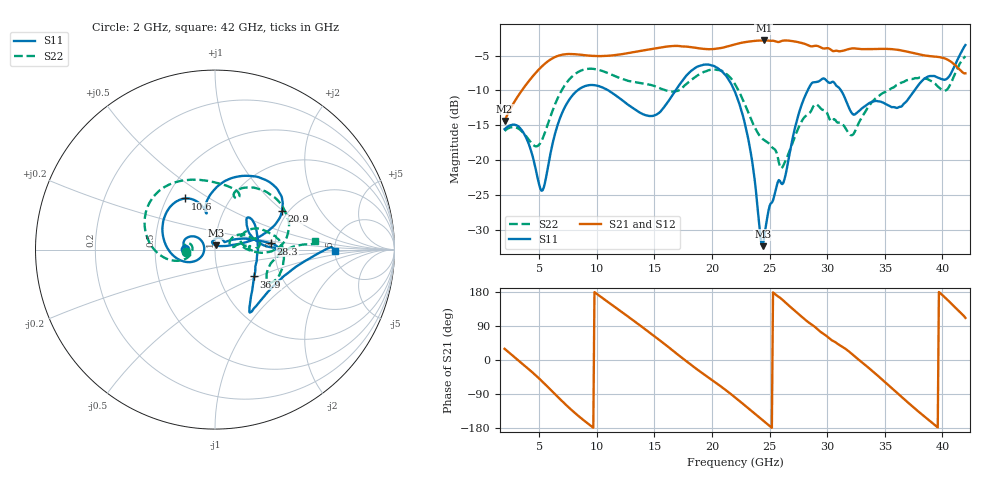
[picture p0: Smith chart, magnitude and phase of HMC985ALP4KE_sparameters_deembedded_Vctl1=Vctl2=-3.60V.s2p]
!s2p File: Measurements: S11, S21, S12, S22
# GHz S dB R 50.0
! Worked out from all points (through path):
!   401 points, 2 GHz to 42 GHz, reference 50 ohm
!   highest |S21| = -2.83 dB at 24.5 GHz (marker M1); lowest = -14.4 dB at 2 GHz (marker M2)
!   lowest |S11| = -32.4 dB at 24.4 GHz (marker M3), VSWR 1.05, Z = 50.3 + j2.39 ohm
!   |S11| at or under -10 dB: start of sweep to 8.328 GHz; 21.94 GHz to 28.31 GHz (6.371 GHz wide, 25.4 % of centre); 31.2 GHz to 37.58 GHz (6.386 GHz wide, 18.6 % of centre)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
!   |S22| runs from -21.2 to -5.1 dB; largest |S21 - S12| = 0.00067
!   S11 on the Smith chart (normalised r, x): 2 GHz: 0.71, +0.00; 10.6 GHz: 0.62, +0.40; 20.9 GHz: 1.86, +0.98; 28.3 GHz: 1.91, +0.15; 36.9 GHz: 1.47, -0.47; 42 GHz: 5.05, -0.13
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2  -15.57 179.7  -14.38 29.5  -14.38 29.5  -15.82 -175.6
3.6  -15.98 153.0  -9.77 -11.2  -9.78 -11.2  -16.06 167.1
5.3  -24.35 -176.9  -6.46 -57.7  -6.45 -57.7  -16.91 -167.3
6.9  -13.59 -164.6  -4.91 -105.9  -4.91 -105.9  -10.15 -174.9
8.7  -9.59 149.6  -4.90 -155.0  -4.90 -155.0  -7.11 150.0
10.6  -9.66 120.0  -5.07 161.3  -5.07 161.2  -7.28 118.9
13.3  -12.72 104.2  -4.48 101.6  -4.48 101.5  -8.80 80.5
15.4  -13.24 104.0  -3.89 53.5  -3.88 53.5  -9.63 65.6
17.9  -7.66 75.7  -3.73 -6.0  -3.73 -6.0  -8.93 68.8
20.9  -7.33 29.8  -3.88 -72.6  -3.89 -72.6  -7.21 18.7
22  -10.22 18.9  -3.39 -98.6  -3.39 -98.6  -9.11 1.4
23.2  -17.39 13.4  -2.99 -128.5  -2.99 -128.5  -13.38 -2.9
24.4  -32.37 81.3  -2.83 -158.7  -2.83 -158.6  -16.98 10.5
24.5  -31.48 94.4  -2.83 -161.2  -2.83 -161.2  -17.10 11.4
26.1  -23.46 39.6  -2.88 159.5  -2.88 159.5  -21.07 23.7
28.3  -10.03 6.2  -3.48 101.2  -3.48 101.2  -13.45 17.7
28.7  -8.91 0.5  -3.68 92.8  -3.68 92.8  -12.62 15.2
32.4  -13.46 29.3  -3.97 9.4  -3.97 9.4  -15.94 25.7
35.4  -12.21 13.8  -4.06 -68.6  -4.05 -68.6  -9.90 16.3
36.9  -11.56 -34.4  -4.42 -109.1  -4.42 -109.2  -8.55 3.9
39.6  -8.15 -55.6  -5.19 -178.0  -5.19 -178.0  -9.44 -30.5
42  -3.48 -0.6  -7.55 111.0  -7.55 111.0  -5.08 4.9
